FUNCTION_BLOCK PID_AutoTune
VAR_INPUT
	PV : REAL; // 过程变量（Process Value），即当前温度
	AutoTuneActive : BOOL;
	StepResponseAmplitude : REAL := 20.0; // 阶跃响应的输出幅度
END_VAR
VAR_OUTPUT
	Output 	: REAL; // 控制器输出
    Kp 		: REAL; // 比例增益
    Ki 		: REAL; // 积分增益
    Kd 		: REAL; // 微分增益
	Done	: BOOL;
END_VAR
VAR
    StepResponseStartTime : REAL := 0.0; // 阶跃响应开始时间（以秒为单位）
    StepResponsePVStart : REAL; // 阶跃响应开始时的PV值
    StepResponsePVEnd : REAL; // 阶跃响应结束时的PV值
    StepResponseTime : REAL; // 阶跃响应时间（以秒为单位）
    Ku : REAL; // 临界增益
    Tu : REAL; // 临界周期（以秒为单位）
    // 时间相关变量
    CurrentTime : REAL; // 当前时间（以秒为单位）
	NT_Time:TIME;
	D_Dec:TON;
	monitor:REAL;
END_VAR

	D_Dec(IN:= AutoTuneActive, PT:= T#1600S, Q=> , ET=> NT_Time);	
	CurrentTime := TIME_TO_REAL(NT_Time) / 1000.0; 	// 将毫秒转换为秒
	IF NOT AutoTuneActive 
		THEN 
		StepResponseStartTime := 0.0;	
		IF Done 
			THEN 
			Done := FALSE;
		END_IF;
	END_IF;
	monitor:=StepResponsePVStart + StepResponseAmplitude * 0.63;
	IF AutoTuneActive THEN
		// 开始阶跃响应测试
		IF StepResponseStartTime = 0.0 THEN
			StepResponseStartTime := CurrentTime; 	// 记录开始时间
			StepResponsePVStart := PV; 				// 记录初始PV值
			Output := StepResponseAmplitude;		// 设置阶跃输出
		END_IF
	
		// 等待系统响应
		IF PV >= StepResponsePVStart + StepResponseAmplitude * 0.63 THEN
			StepResponseTime := CurrentTime - StepResponseStartTime; // 计算响应时间
			StepResponsePVEnd := PV; // 记录结束PV值
			AutoTuneActive := FALSE; // 结束自整定
			Done:=TRUE;
	
			Ku := 4 * StepResponseAmplitude / (StepResponsePVEnd - StepResponsePVStart); // 临界增益
			Tu := StepResponseTime; // 临界周期

			Kp := 0.6 * Ku;
			Ki := 1.2 * Ku / Tu;
			Kd := 0.075 * Ku * Tu;
		END_IF
	END_IF

END_FUNCTION_BLOCK
